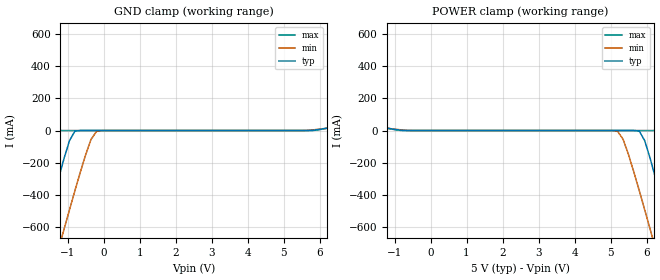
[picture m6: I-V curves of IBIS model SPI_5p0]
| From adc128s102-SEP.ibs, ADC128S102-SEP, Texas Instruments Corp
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|   Model SPI_5p0
[Model]  SPI_5p0
Model_type Input
Vinl = 0
Vinh = 5.0
C_comp   100.8fF   99.7fF   101.6fF
[Temperature Range]   25.0000   105.00   -40.00
[Voltage Range]   5.0V   4.50V   5.50V
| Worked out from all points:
|   GND clamp passes 1 mA (typ) near -0.68 V on its own axis
|   POWER clamp passes 1 mA (typ) near -0.75 V on its own axis
[Power Clamp]
|Voltage   I(typ)   I(min)   I(max)
-5V       1.95A      1.81A      2.11A
-2.9V     701mA      720mA      687mA
-2.75V    613mA      643mA      587mA
-2V       183mA      265mA      102mA
-1.55V    27.6mA     58mA       31mA
5.2V      -13.2pA    -5.65mA    -9.65pA
5.8V      -4.3mA     -376mA     -12.2pA
6.1V      -174mA     -615mA     -8.85nA
6.4V      -423mA     -857mA     -5.69mA
6.7V      -684mA     -1.1A      -215mA
7.15V     -1.08A     -1.47A     -630mA
10V       -3.64A     -3.85A     -3.37A
[Gnd Clamp]
|Voltage   I(typ)   I(min)   I(max)
-5V       -3.64A     -3.85A     -3.37A
-2.15V    -1.08A     -1.47A     -630mA
-1.7V     -684mA     -1.1A      -215mA
-1.4V     -423mA     -857mA     -5.69mA
-1.1V     -174mA     -615mA     -8.85nA
-800mV    -4.3mA     -376mA     -12.2pA
-200mV    -13.2pA    -5.65mA    -9.65pA
6.55V     27.6mA     58mA       31mA
7V        183mA      265mA      102mA
7.75V     613mA      643mA      587mA
7.9V      701mA      720mA      687mA
10V       1.95A      1.81A      2.11A
